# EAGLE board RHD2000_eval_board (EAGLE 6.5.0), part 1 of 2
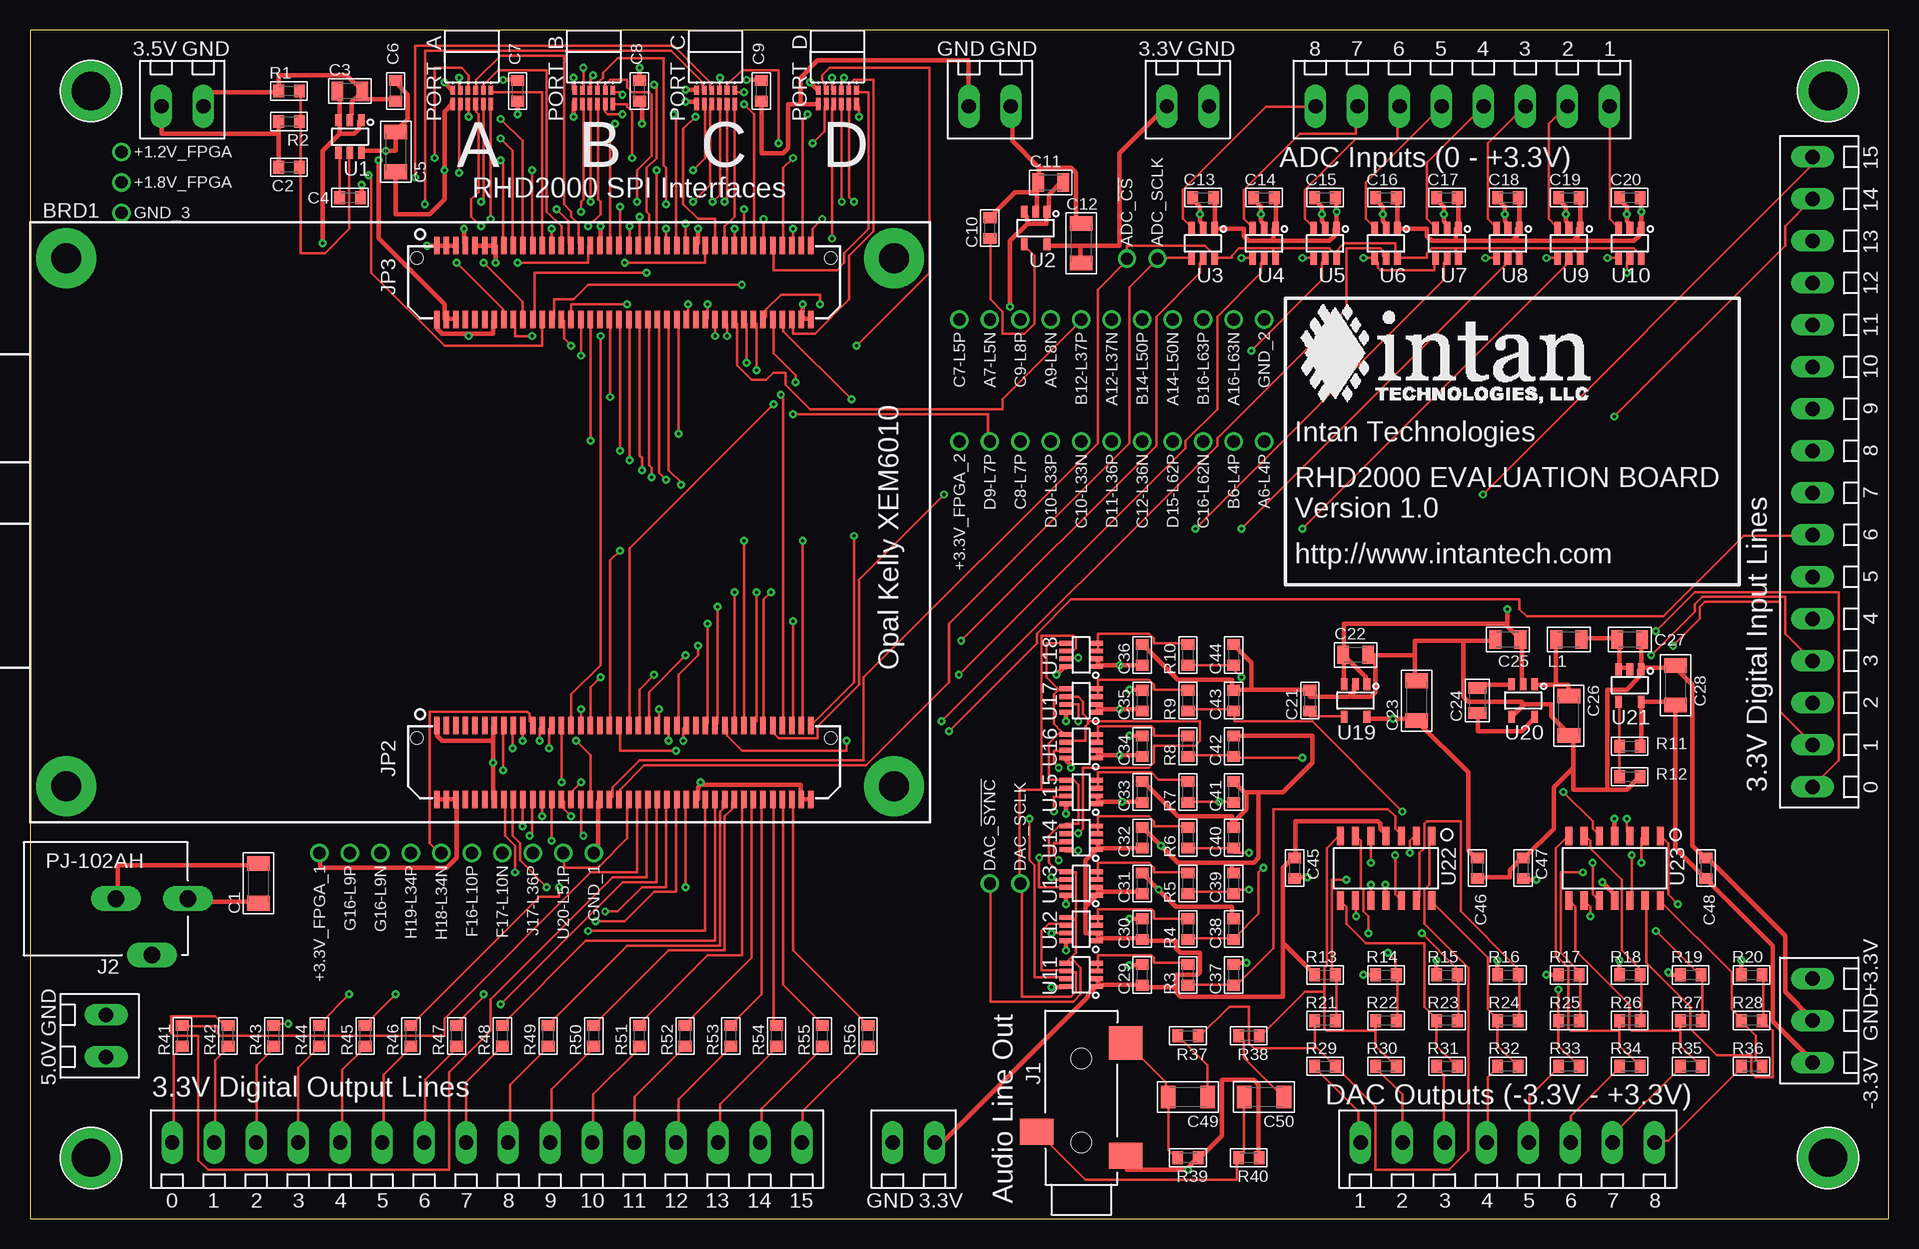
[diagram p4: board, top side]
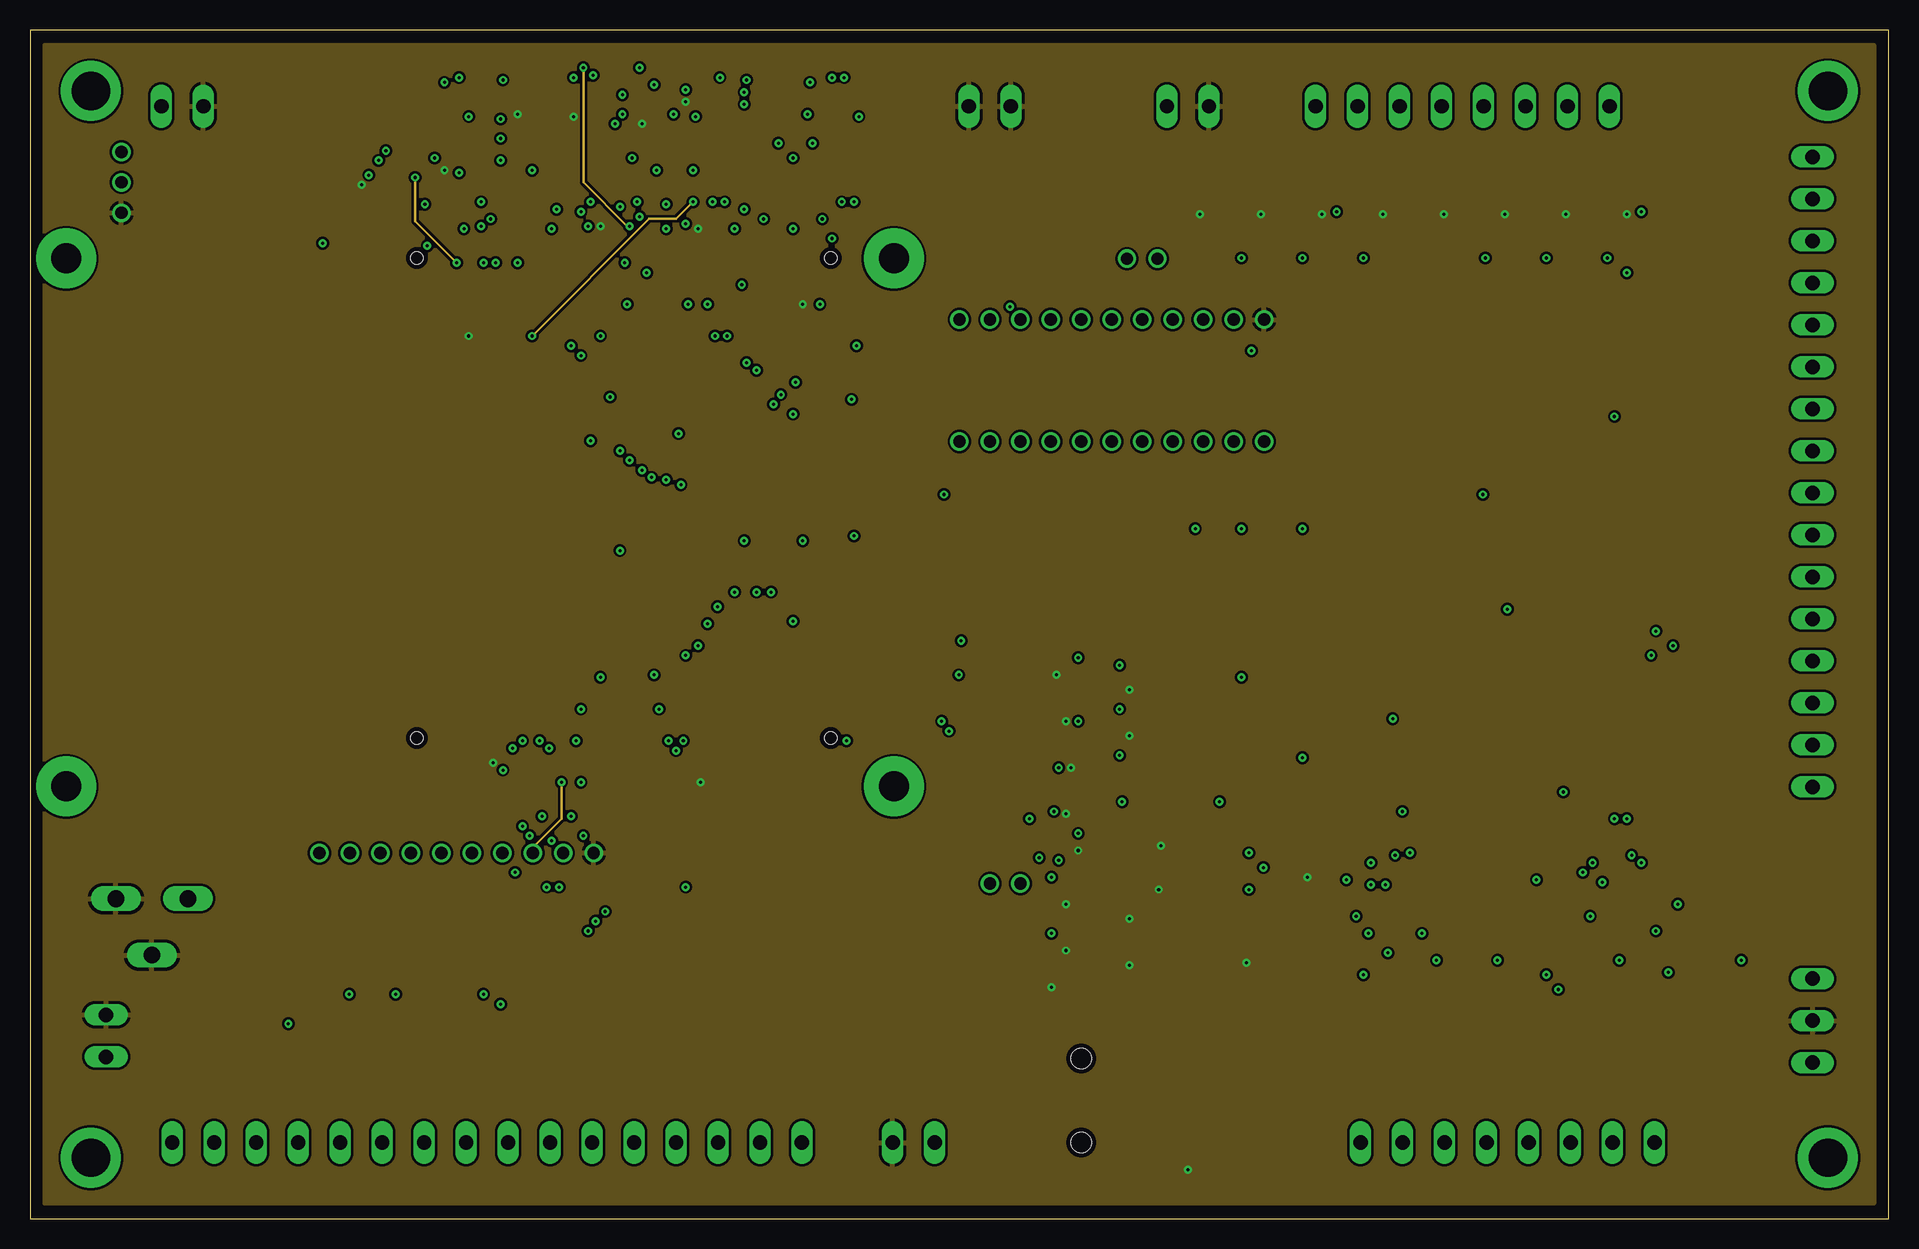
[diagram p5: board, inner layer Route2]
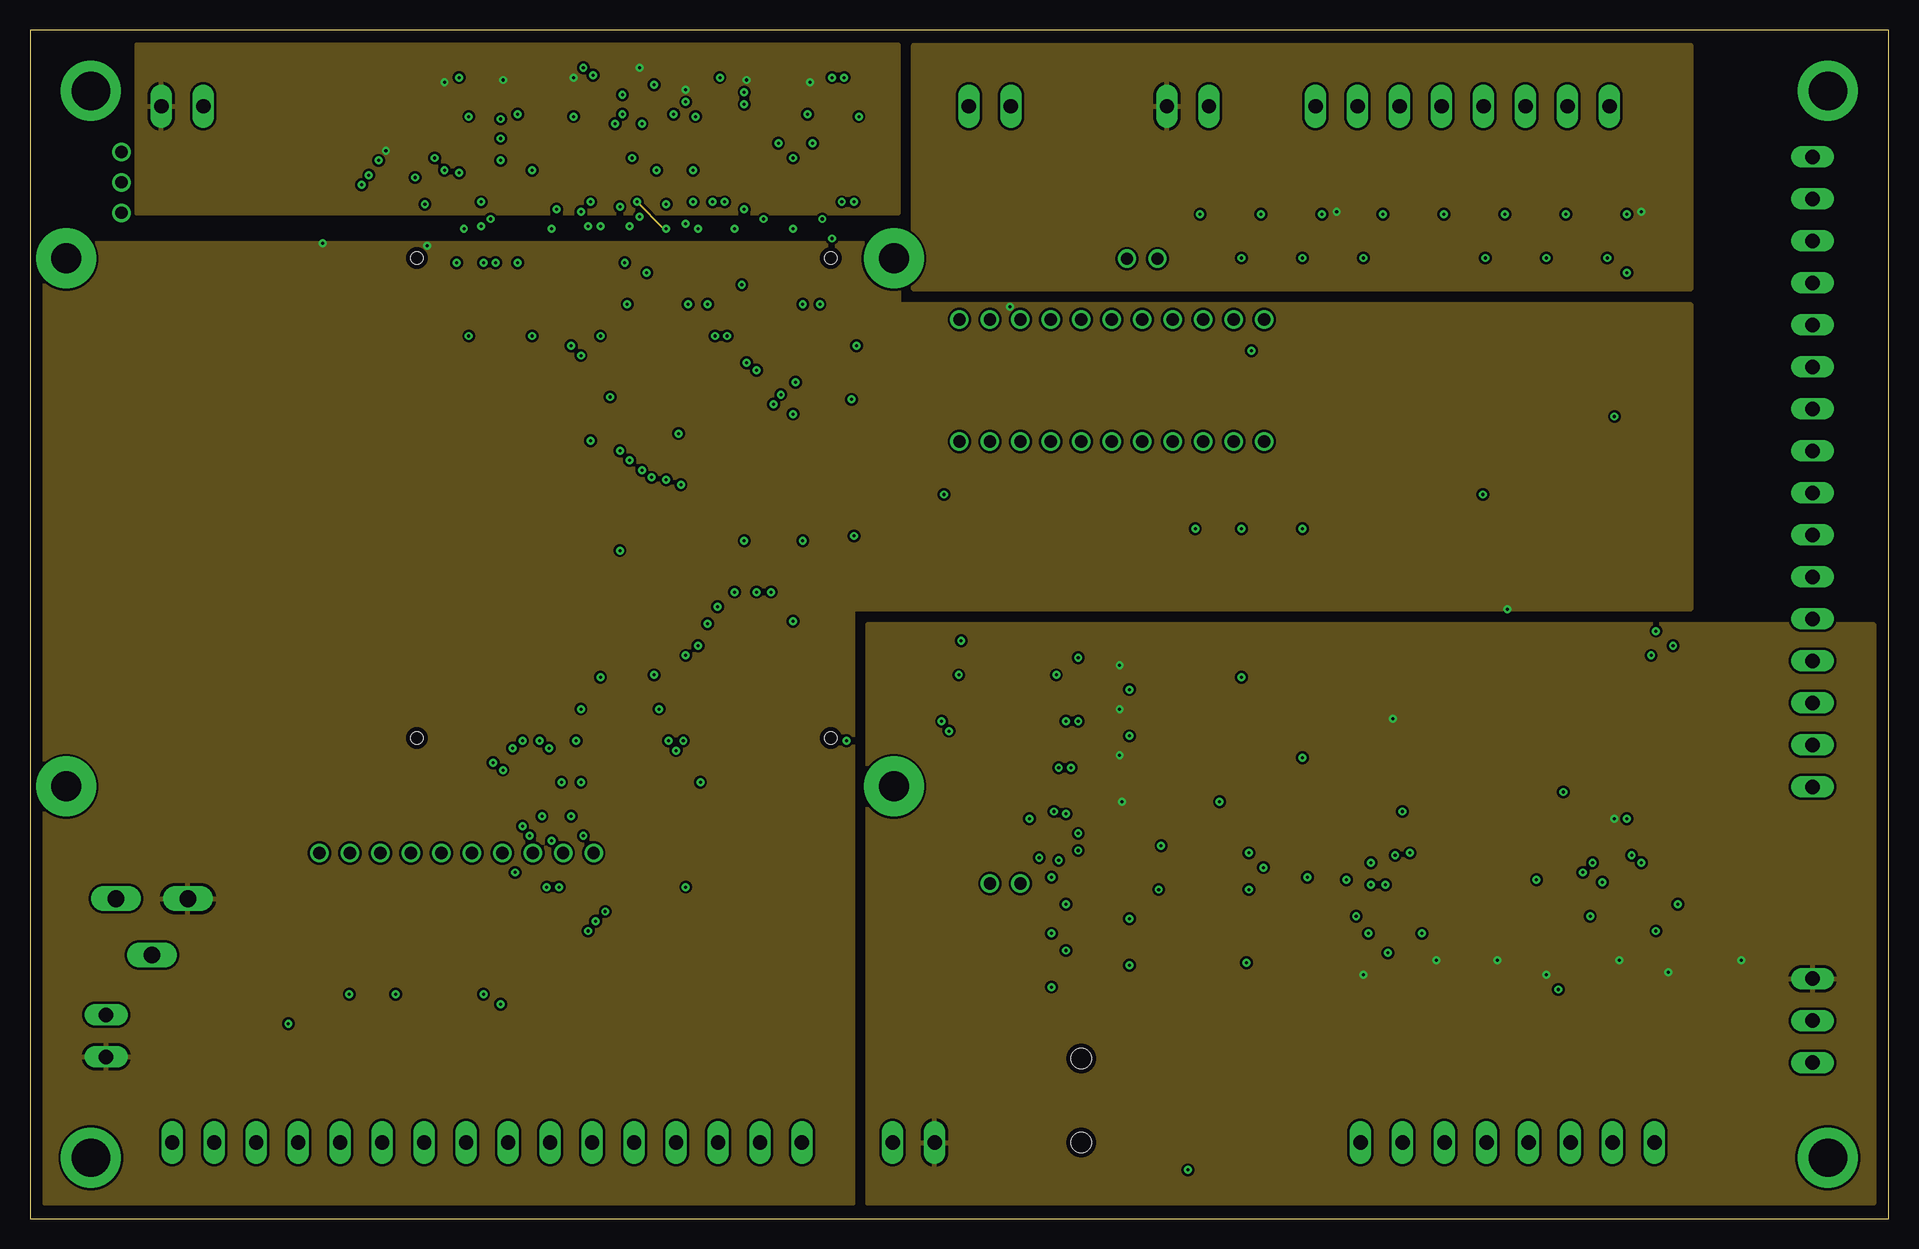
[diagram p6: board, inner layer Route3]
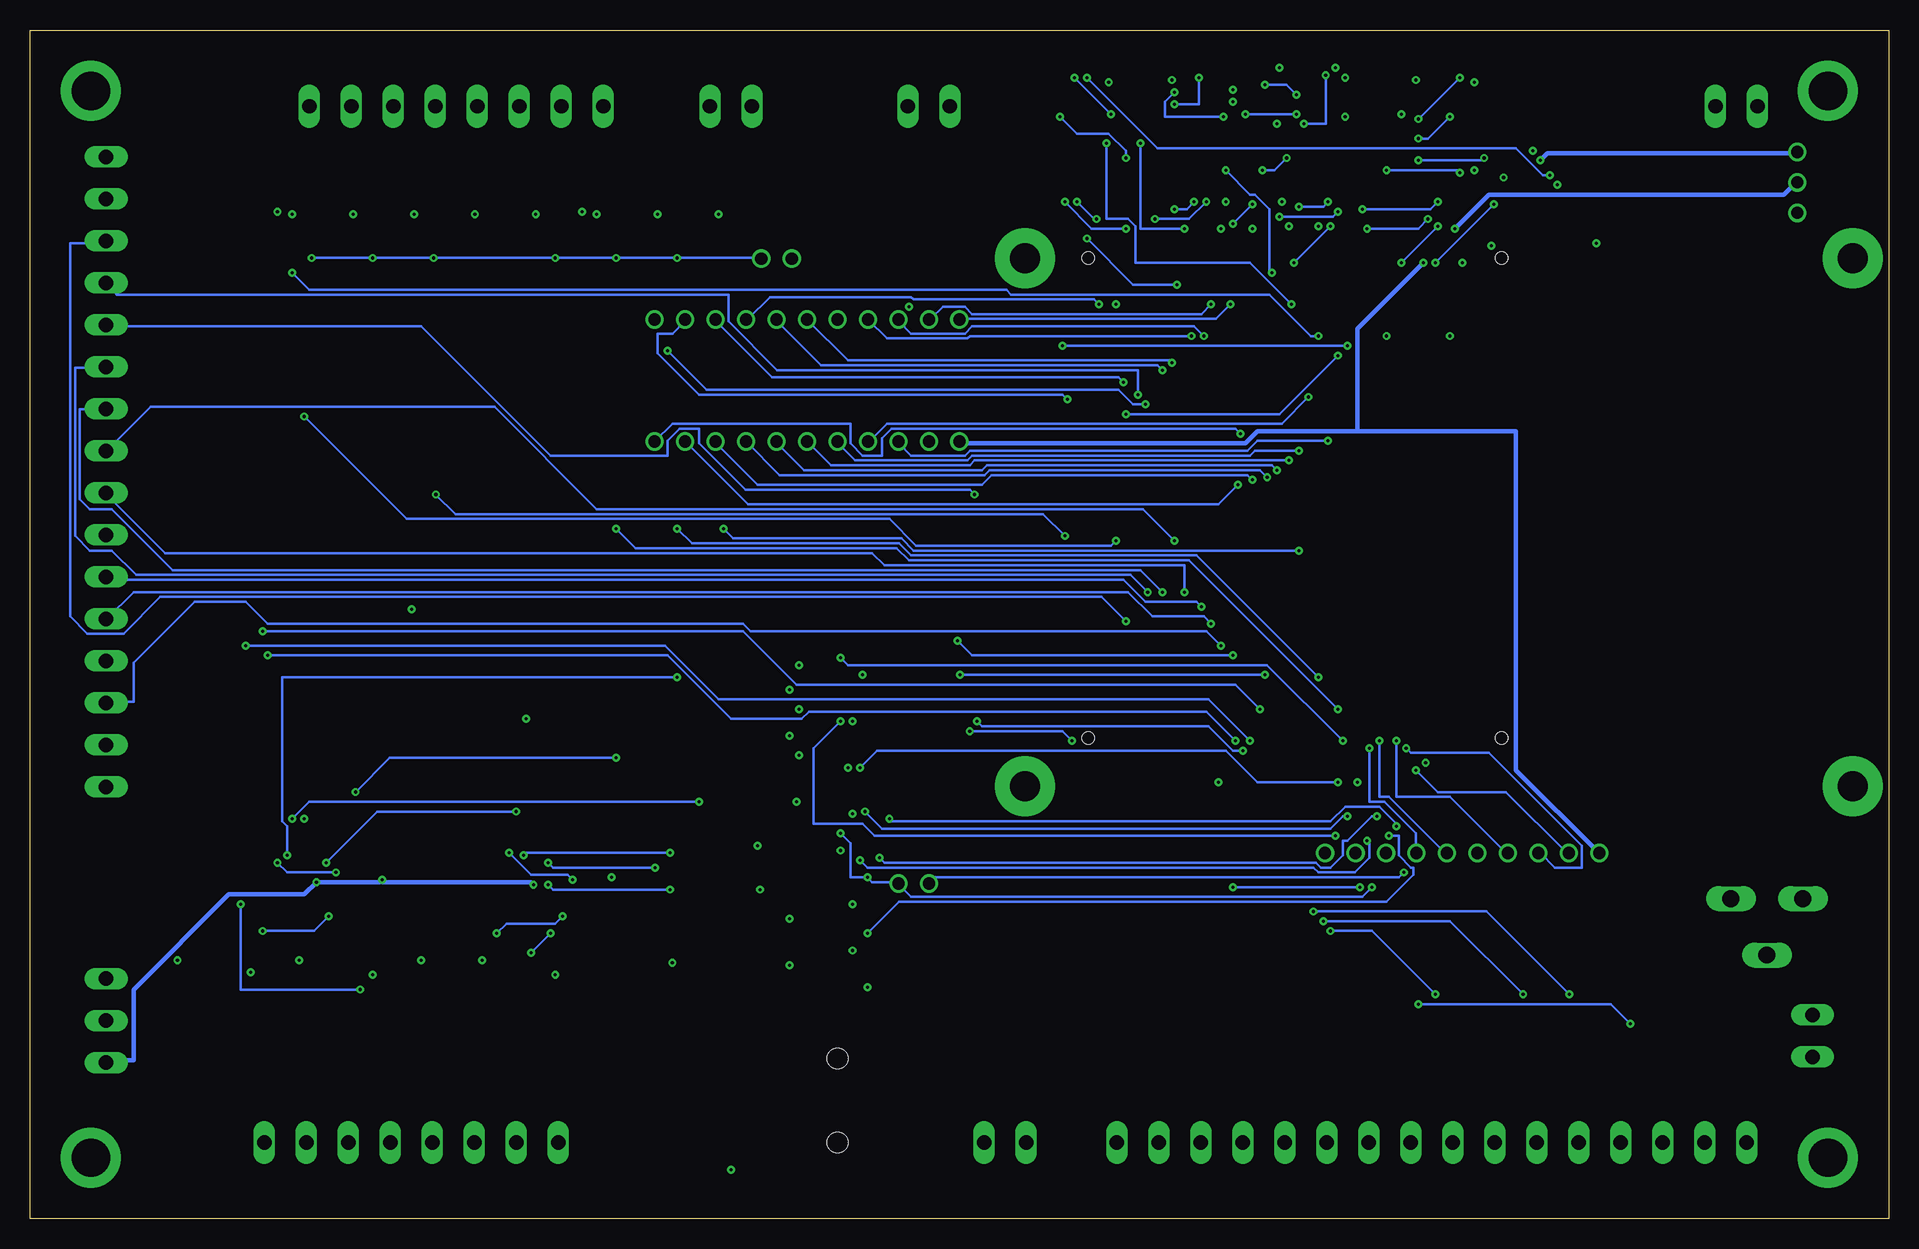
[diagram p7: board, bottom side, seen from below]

Size 154.94 x 99.06 mm. Coordinates in mm from the lower left corner, seen from the top.
Outline: 0,0 154.94,0 154.94,99.06 0,99.06 0,0
Copper layers (1*2+3*16): Top 0.035mm / dielectric 1.5mm / Route2 0.035mm / dielectric 0.15mm / Route3 0.035mm / dielectric 0.2mm / Bottom 0.035mm
Design rules "default": minimum track width 8mil, minimum drill 10mil, track to track 8mil, track to pad 8mil, pad to pad 8mil, via to via 8mil, smd to smd 8mil, copper to edge 15mil, drill to drill 8mil, minimum pad ring 10mil, minimum via ring 8mil, stop-mask expansion 4mil, vias tented up to drill 0mil, thermal gap 10mil
Net classes: 1 power: width 0.381 mm
tRestrict: area 141,33 to 154.9,34.3; area 139.7,33 to 141,50.8; area 137.2,78.7 to 138.4,99.1
vRestrict: area 36.8,85.1 to 68.6,86.9; area 105.4,54.6 to 137.2,56.4; area 105.4,64.8 to 130.8,66.5; area 105.4,61 to 142.2,62.7; area 35.6,87.6 to 38.1,91.4; area 45.7,87.6 to 48.3,91.4; area 55.9,87.6 to 58.4,91.4; area 66,87.6 to 68.6,91.4; area 105.4,58.4 to 120.7,60.2; area 105.7,67.8 to 130.3,76.2

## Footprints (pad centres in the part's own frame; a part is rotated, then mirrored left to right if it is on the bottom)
TERMINAL_BLOCK_3.5MM_16 = drill 1.2 long: 1 -26.25,0; 2 -22.75,0; 3 -19.25,0; 4 -15.75,0; 5 -12.25,0; 6 -8.75,0; 7 -5.25,0; 8 -1.75,0; 9 1.75,0; 10 5.25,0; 11 8.75,0; 12 12.25,0; 13 15.75,0; 14 19.25,0; 15 22.75,0; 16 26.25,0
TESTPOINT = drill 1.016: 1 0,0
TERMINAL_BLOCK_3.5MM_8 = drill 1.2 long: 1 -12.28,0; 2 -8.78,0; 3 -5.28,0; 4 -1.78,0; 5 1.72,0; 6 5.22,0; 7 8.72,0; 8 12.22,0
OPALKELLY_XEM6010 = drill 2.5 pad 5: HOLE_NC_1 3,3; HOLE_NC_2 3,47; HOLE_NC_3 72,3; HOLE_NC_4 72,47 | smd 0.457 x 1.448: JP2-1 33.9,8.086; JP2-2 33.9,1.914; JP2-3 34.7,8.086; JP2-4 34.7,1.914; JP2-5 35.5,8.086; JP2-6 35.5,1.914; JP2-7 36.3,8.086; JP2-8 36.3,1.914; JP2-9 37.1,8.086; JP2-10 37.1,1.914; JP2-11 37.9,8.086; JP2-12 37.9,1.914; JP2-13 38.7,8.086; JP2-14 38.7,1.914; JP2-15 39.5,8.086; JP2-16 39.5,1.914; JP2-17 40.3,8.086; JP2-18 40.3,1.914; JP2-19 41.1,8.086; JP2-20 41.1,1.914; JP2-21 41.9,8.086; JP2-22 41.9,1.914; JP2-23 42.7,8.086; JP2-24 42.7,1.914; JP2-25 43.5,8.086; JP2-26 43.5,1.914; JP2-27 44.3,8.086; JP2-28 44.3,1.914; JP2-29 45.1,8.086; JP2-30 45.1,1.914; JP2-31 45.9,8.086; JP2-32 45.9,1.914; JP2-33 46.7,8.086; JP2-34 46.7,1.914; JP2-35 47.5,8.086; JP2-36 47.5,1.914; JP2-37 48.3,8.086; JP2-38 48.3,1.914; JP2-39 49.1,8.086; JP2-40 49.1,1.914; JP2-41 49.9,8.086; JP2-42 49.9,1.914; JP2-43 50.7,8.086; JP2-44 50.7,1.914; JP2-45 51.5,8.086; JP2-46 51.5,1.914; JP2-47 52.3,8.086; JP2-48 52.3,1.914; JP2-49 53.1,8.086; JP2-50 53.1,1.914; JP2-51 53.9,8.086; JP2-52 53.9,1.914; JP2-53 54.7,8.086; JP2-54 54.7,1.914; JP2-55 55.5,8.086; JP2-56 55.5,1.914; JP2-57 56.3,8.086; JP2-58 56.3,1.914; JP2-59 57.1,8.086; JP2-60 57.1,1.914; JP2-61 57.9,8.086; JP2-62 57.9,1.914; JP2-63 58.7,8.086; JP2-64 58.7,1.914; JP2-65 59.5,8.086; JP2-66 59.5,1.914; JP2-67 60.3,8.086; JP2-68 60.3,1.914; JP2-69 61.1,8.086; JP2-70 61.1,1.914; JP2-71 61.9,8.086; JP2-72 61.9,1.914; JP2-73 62.7,8.086; JP2-74 62.7,1.914; JP2-75 63.5,8.086; JP2-76 63.5,1.914; JP2-77 64.3,8.086; JP2-78 64.3,1.914; JP2-79 65.1,8.086; JP2-80 65.1,1.914; JP3-1 33.9,48.086; JP3-2 33.9,41.914; JP3-3 34.7,48.086; JP3-4 34.7,41.914; JP3-5 35.5,48.086; JP3-6 35.5,41.914; JP3-7 36.3,48.086; JP3-8 36.3,41.914; JP3-9 37.1,48.086; JP3-10 37.1,41.914; JP3-11 37.9,48.086; JP3-12 37.9,41.914; JP3-13 38.7,48.086; JP3-14 38.7,41.914; JP3-15 39.5,48.086; JP3-16 39.5,41.914; JP3-17 40.3,48.086; JP3-18 40.3,41.914; JP3-19 41.1,48.086; JP3-20 41.1,41.914; JP3-21 41.9,48.086; JP3-22 41.9,41.914; JP3-23 42.7,48.086; JP3-24 42.7,41.914; JP3-25 43.5,48.086; JP3-26 43.5,41.914; JP3-27 44.3,48.086; JP3-28 44.3,41.914; JP3-29 45.1,48.086; JP3-30 45.1,41.914; JP3-31 45.9,48.086; JP3-32 45.9,41.914; JP3-33 46.7,48.086; JP3-34 46.7,41.914; JP3-35 47.5,48.086; JP3-36 47.5,41.914; JP3-37 48.3,48.086; JP3-38 48.3,41.914; JP3-39 49.1,48.086; JP3-40 49.1,41.914; JP3-41 49.9,48.086; JP3-42 49.9,41.914; JP3-43 50.7,48.086; JP3-44 50.7,41.914; JP3-45 51.5,48.086; JP3-46 51.5,41.914; JP3-47 52.3,48.086; JP3-48 52.3,41.914; JP3-49 53.1,48.086; JP3-50 53.1,41.914; JP3-51 53.9,48.086; JP3-52 53.9,41.914; JP3-53 54.7,48.086; JP3-54 54.7,41.914; JP3-55 55.5,48.086; JP3-56 55.5,41.914; JP3-57 56.3,48.086; JP3-58 56.3,41.914; JP3-59 57.1,48.086; JP3-60 57.1,41.914; JP3-61 57.9,48.086; JP3-62 57.9,41.914; JP3-63 58.7,48.086; JP3-64 58.7,41.914; JP3-65 59.5,48.086; JP3-66 59.5,41.914; JP3-67 60.3,48.086; JP3-68 60.3,41.914; JP3-69 61.1,48.086; JP3-70 61.1,41.914; JP3-71 61.9,48.086; JP3-72 61.9,41.914; JP3-73 62.7,48.086; JP3-74 62.7,41.914; JP3-75 63.5,48.086; JP3-76 63.5,41.914; JP3-77 64.3,48.086; JP3-78 64.3,41.914; JP3-79 65.1,48.086; JP3-80 65.1,41.914 | hole 1.016: 32.261,47.032; 66.739,47.032; 32.261,7.032; 66.739,7.032
1206 = smd 1.219 x 1.88: 1 -1.651,0; 2 1.651,0
0603 = smd 0.889 x 1.067: 1 -0.864,0; 2 0.864,0
0805 = smd 0.965 x 1.524: 1 -1.041,0; 2 1.041,0
SCREW_HOLE_4-40 = drill 3.2 pad 5: 1 0,0
SJ-3523 = smd 2.2 x 2.8: 1 -1.1,-3.7; 3 0.9,3.7 | smd 2.8 x 2.8: 2 8.3,-3.7 | hole 1.7: 7,0; 0,0
PJ-102AH = drill 1.4 long: 1 0,-3; 2 0,3; 3 -4.7,0
OMNETICS_PZN-12-AA = smd 0.381 x 0.762: B1 1.587,-1.016; B2 0.953,-1.016; B3 0.318,-1.016; B4 -0.318,-1.016; B5 -0.953,-1.016; B6 -1.587,-1.016 | smd 0.381 x 1.016: T1 1.587,-2.159; T2 0.953,-2.159; T3 0.318,-2.159; T4 -0.318,-2.159; T5 -0.953,-2.159; T6 -1.587,-2.159
TERMINAL_BLOCK_3.5MM_3 = drill 1.2 long: + 3.5,0; - -3.5,0; GND 0,0
TERMINAL_BLOCK_3.5MM_2_3.3V = drill 1.2 long: 1 -1.75,0; 2 1.75,0
TERMINAL_BLOCK_3.5MM_2_GND = drill 1.2 long: 1 -1.75,0; 2 1.75,0
TERMINAL_BLOCK_3.5MM_2_5V = drill 1.2 long: 1 -1.75,0; 2 1.75,0
TERMINAL_BLOCK_3.5MM_2_3.5V = drill 1.2 long: 1 -1.75,0; 2 1.75,0
SOT-23-6 = smd 0.55 x 1: 1 -0.95,-1.35; 2 0,-1.35; 3 0.95,-1.35; 4 0.95,1.35; 5 0,1.35; 6 -0.95,1.35
SOT-23-5 = smd 0.55 x 1: 1 -0.95,-1.35; 2 0,-1.35; 3 0.95,-1.35; 4 0.95,1.35; 5 -0.95,1.35
SOT-23-RJ-6 = smd 0.55 x 1: 1 -0.95,-1.3; 2 0,-1.3; 3 0.95,-1.3; 4 0.95,1.3; 5 0,1.3; 6 -0.95,1.3
SOT-23-RJ-8 = smd 0.4 x 1: 1 -0.975,-1.3; 2 -0.325,-1.3; 3 0.325,-1.3; 4 0.975,-1.3; 5 0.975,1.3; 6 0.325,1.3; 7 -0.325,1.3; 8 -0.975,1.3
SOIC-14 = smd 0.6 x 1.55: 1 -3.81,-2.7; 2 -2.54,-2.7; 3 -1.27,-2.7; 4 0,-2.7; 5 1.27,-2.7; 6 2.54,-2.7; 7 3.81,-2.7; 8 3.81,2.7; 9 2.54,2.7; 10 1.27,2.7; 11 0,2.7; 12 -1.27,2.7; 13 -2.54,2.7; 14 -3.81,2.7

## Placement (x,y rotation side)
3.3V_DIGITAL_IN  TERMINAL_BLOCK_16-3.5MM  [TERMINAL_BLOCK_3.5MM_16]  148.59,62.23 90 top
3.3V_DIGITAL_OUT  TERMINAL_BLOCK_16-3.5MM  [TERMINAL_BLOCK_3.5MM_16]  38.1,6.35 0 top
+1.2V_FPGA  TESTPOINT  [TESTPOINT]  7.62,88.9 0 top
+1.8V_FPGA  TESTPOINT  [TESTPOINT]  7.62,86.36 0 top
+3.3V_FPGA_1  TESTPOINT  [TESTPOINT]  24.13,30.48 270 top
+3.3V_FPGA_2  TESTPOINT  [TESTPOINT]  77.47,64.77 270 top
A6-L4P  TESTPOINT  [TESTPOINT]  102.87,64.77 270 top
A7-L5N  TESTPOINT  [TESTPOINT]  80.01,74.93 270 top
A9-L8N  TESTPOINT  [TESTPOINT]  85.09,74.93 270 top
A12-L37N  TESTPOINT  [TESTPOINT]  90.17,74.93 270 top
A14-L50N  TESTPOINT  [TESTPOINT]  95.25,74.93 270 top
A16-L63N  TESTPOINT  [TESTPOINT]  100.33,74.93 270 top
ADC_!CS!  TESTPOINT  [TESTPOINT]  91.44,80.01 90 top
ADC_IN  TERMINAL_BLOCK_8-3.5MM  [TERMINAL_BLOCK_3.5MM_8]  119.38,92.71 180 top
ADC_SCLK  TESTPOINT  [TESTPOINT]  93.98,80.01 90 top
B6-L4P  TESTPOINT  [TESTPOINT]  100.33,64.77 270 top
B12-L37P  TESTPOINT  [TESTPOINT]  87.63,74.93 270 top
B14-L50P  TESTPOINT  [TESTPOINT]  92.71,74.93 270 top
B16-L63P  TESTPOINT  [TESTPOINT]  97.79,74.93 270 top
BRD1  OPALKELLY_XEM6010  [OPALKELLY_XEM6010]  0,33.02 0 top
C1  22u  [1206]  19.05,27.94 90 top
C2  15p  [0603]  21.59,87.63 0 top
C3  1.0u  [0805]  26.67,93.98 0 top
C4  10n  [0603]  26.67,85.09 0 top
C5  22u  [1206]  30.48,88.9 270 top
C6  100n  [0603]  30.48,93.98 270 top
C7  100n  [0603]  40.64,93.98 270 top
C7-L5P  TESTPOINT  [TESTPOINT]  77.47,74.93 270 top
C8  100n  [0603]  50.8,93.98 270 top
C8-L7P  TESTPOINT  [TESTPOINT]  82.55,64.77 270 top
C9  100n  [0603]  60.96,93.98 270 top
C9-L8P  TESTPOINT  [TESTPOINT]  82.55,74.93 270 top
C10  10n  [0603]  80.01,82.55 90 top
C10-L33N  TESTPOINT  [TESTPOINT]  87.63,64.77 270 top
C11  1.0u  [0805]  85.09,86.36 180 top
C12  22u  [1206]  87.63,81.28 90 top
C12-L36N  TESTPOINT  [TESTPOINT]  92.71,64.77 270 top
C13  100n  [0603]  97.79,85.09 180 top
C14  100n  [0603]  102.87,85.09 180 top
C15  100n  [0603]  107.95,85.09 180 top
C16  100n  [0603]  113.03,85.09 180 top
C16-L62N  TESTPOINT  [TESTPOINT]  97.79,64.77 270 top
C17  100n  [0603]  118.11,85.09 180 top
C18  100n  [0603]  123.19,85.09 180 top
C19  100n  [0603]  128.27,85.09 180 top
C20  100n  [0603]  133.35,85.09 180 top
C21  10n  [0603]  106.68,43.18 90 top
C22  1.0u  [0805]  110.49,46.99 0 top
C23  22u  [1206]  115.57,43.18 90 top
C24  1.0u  [0805]  120.65,43.18 90 top
C25  1.0u  [0805]  123.19,48.26 180 top
C26  10u  [1206]  128.27,41.91 270 top
C27  1.0u  [0805]  133.35,48.26 0 top
C28  22u  [1206]  137.16,44.45 90 top
C29  100n  [0603]  92.71,20.32 90 top
C30  100n  [0603]  92.71,24.13 90 top
C31  100n  [0603]  92.71,27.94 90 top
C32  100n  [0603]  92.71,31.75 90 top
C33  100n  [0603]  92.71,35.56 90 top
C34  100n  [0603]  92.71,39.37 90 top
C35  100n  [0603]  92.71,43.18 90 top
C36  100n  [0603]  92.71,46.99 90 top
C37  1n  [0603]  100.33,20.32 90 top
C38  1n  [0603]  100.33,24.13 90 top
C39  1n  [0603]  100.33,27.94 90 top
C40  1n  [0603]  100.33,31.75 90 top
C41  1n  [0603]  100.33,35.56 90 top
C42  1n  [0603]  100.33,39.37 90 top
C43  1n  [0603]  100.33,43.18 90 top
C44  1n  [0603]  100.33,46.99 90 top
C45  100n  [0603]  105.41,29.21 270 top
C46  100n  [0603]  120.65,29.21 270 top
C47  100n  [0603]  124.46,29.21 270 top
C48  100n  [0603]  139.7,29.21 270 top
C49  22u  [1206]  96.52,10.16 180 top
C50  22u  [1206]  102.87,10.16 180 top
D9-L7P  TESTPOINT  [TESTPOINT]  80.01,64.77 270 top
D10-L33P  TESTPOINT  [TESTPOINT]  85.09,64.77 270 top
D11-L36P  TESTPOINT  [TESTPOINT]  90.17,64.77 270 top
D15-L62P  TESTPOINT  [TESTPOINT]  95.25,64.77 270 top
DAC_!SYNC!  TESTPOINT  [TESTPOINT]  80.01,27.94 90 top
DAC_OUT  TERMINAL_BLOCK_8-3.5MM  [TERMINAL_BLOCK_3.5MM_8]  123.19,6.35 0 top
DAC_SCLK  TESTPOINT  [TESTPOINT]  82.55,27.94 90 top
F16-L10P  TESTPOINT  [TESTPOINT]  36.83,30.48 270 top
F17-L10N  TESTPOINT  [TESTPOINT]  39.37,30.48 270 top
G16-L9N  TESTPOINT  [TESTPOINT]  29.21,30.48 270 top
G16-L9P  TESTPOINT  [TESTPOINT]  26.67,30.48 270 top
GND_1  TESTPOINT  [TESTPOINT]  46.99,30.48 270 top
GND_2  TESTPOINT  [TESTPOINT]  102.87,74.93 270 top
GND_3  TESTPOINT  [TESTPOINT]  7.62,83.82 0 top
H1  SCREW_HOLE_4-40  [SCREW_HOLE_4-40]  5.08,93.98 0 top
H2  SCREW_HOLE_4-40  [SCREW_HOLE_4-40]  149.86,93.98 0 top
H3  SCREW_HOLE_4-40  [SCREW_HOLE_4-40]  149.86,5.08 0 top
H4  SCREW_HOLE_4-40  [SCREW_HOLE_4-40]  5.08,5.08 0 top
H18-L34N  TESTPOINT  [TESTPOINT]  34.29,30.48 270 top
H19-L34P  TESTPOINT  [TESTPOINT]  31.75,30.48 270 top
J1  STEREO_JACK_SJ-3523  [SJ-3523]  87.63,6.35 90 top
J2  DC_POWER_JACK-PJ-102AH  [PJ-102AH]  10.16,26.67 90 top
J17-L36P  TESTPOINT  [TESTPOINT]  41.91,30.48 270 top
L1  100n  [0805]  128.27,48.26 0 top
LOGO1  INTAN_LOGO  [INTAN_LOGO]  105.41,67.31 0 top
PORT_A  RHD2000-CABLE-DAQ-SIDE  [OMNETICS_PZN-12-AA]  36.83,95.05 0 top
PORT_B  RHD2000-CABLE-DAQ-SIDE  [OMNETICS_PZN-12-AA]  46.99,95.05 0 top
PORT_C  RHD2000-CABLE-DAQ-SIDE  [OMNETICS_PZN-12-AA]  57.15,95.05 0 top
PORT_D  RHD2000-CABLE-DAQ-SIDE  [OMNETICS_PZN-12-AA]  67.31,95.05 0 top
R1  30.1K  [0603]  21.59,93.98 0 top
R2  56.0K  [0603]  21.59,91.44 180 top
R3  5.6K  [0603]  96.52,20.32 90 top
R4  5.6K  [0603]  96.52,24.13 90 top
R5  5.6K  [0603]  96.52,27.94 90 top
R6  5.6K  [0603]  96.52,31.75 90 top
R7  5.6K  [0603]  96.52,35.56 90 top
R8  5.6K  [0603]  96.52,39.37 90 top
R9  5.6K  [0603]  96.52,43.18 90 top
R10  5.6K  [0603]  96.52,46.99 90 top
R11  64.9K  [0603]  133.35,39.37 0 top
R12  36.0K  [0603]  133.35,36.83 180 top
R13  10k  [0603]  107.95,20.32 0 top
R14  10k  [0603]  113.03,20.32 0 top
R15  10k  [0603]  118.11,20.32 0 top
R16  10k  [0603]  123.19,20.32 0 top
R17  10k  [0603]  128.27,20.32 0 top
R18  10k  [0603]  133.35,20.32 0 top
R19  10k  [0603]  138.43,20.32 0 top
R20  10k  [0603]  143.51,20.32 0 top
R21  10k  [0603]  107.95,16.51 0 top
R22  10k  [0603]  113.03,16.51 0 top
R23  10k  [0603]  118.11,16.51 0 top
R24  10k  [0603]  123.19,16.51 0 top
R25  10k  [0603]  128.27,16.51 0 top
R26  10k  [0603]  133.35,16.51 0 top
R27  10k  [0603]  138.43,16.51 0 top
R28  10k  [0603]  143.51,16.51 0 top
R29  51  [0603]  107.95,12.7 0 top
R30  51  [0603]  113.03,12.7 0 top
R31  51  [0603]  118.11,12.7 0 top
R32  51  [0603]  123.19,12.7 0 top
R33  51  [0603]  128.27,12.7 0 top
R34  51  [0603]  133.35,12.7 0 top
R35  51  [0603]  138.43,12.7 0 top
R36  51  [0603]  143.51,12.7 0 top
R37  100  [0603]  96.52,15.24 180 top
R38  100  [0603]  101.6,15.24 180 top
R39  1.0M  [0603]  96.52,5.08 180 top
R40  1.0M  [0603]  101.6,5.08 180 top
R41  51  [0603]  12.7,15.24 90 top
R42  51  [0603]  16.51,15.24 90 top
R43  51  [0603]  20.32,15.24 90 top
R44  51  [0603]  24.13,15.24 90 top
R45  51  [0603]  27.94,15.24 90 top
R46  51  [0603]  31.75,15.24 90 top
R47  51  [0603]  35.56,15.24 90 top
R48  51  [0603]  39.37,15.24 90 top
R49  51  [0603]  43.18,15.24 90 top
R50  51  [0603]  46.99,15.24 90 top
R51  51  [0603]  50.8,15.24 90 top
R52  51  [0603]  54.61,15.24 90 top
R53  51  [0603]  58.42,15.24 90 top
R54  51  [0603]  62.23,15.24 90 top
R55  51  [0603]  66.04,15.24 90 top
R56  51  [0603]  69.85,15.24 90 top
S1  TERMINAL_BLOCK_3_+/-3.3V  [TERMINAL_BLOCK_3.5MM_3]  148.59,16.51 90 top
S2  TERMINAL_BLOCK_2-3.5MM-3.3V  [TERMINAL_BLOCK_3.5MM_2_3.3V]  96.52,92.71 180 top
S6  TERMINAL_BLOCK_2-3.5MM-3.3V  [TERMINAL_BLOCK_3.5MM_2_3.3V]  73.66,6.35 0 top
S8  TERMINAL_BLOCK_2-3.5MM-GND  [TERMINAL_BLOCK_3.5MM_2_GND]  80.01,92.71 180 top
S9  TERMINAL_BLOCK_2-3.5MM-5V  [TERMINAL_BLOCK_3.5MM_2_5V]  6.35,15.24 270 top
S10  TERMINAL_BLOCK_2-3.5MM-3.5V  [TERMINAL_BLOCK_3.5MM_2_3.5V]  12.7,92.71 180 top
U1  TPS79301  [SOT-23-6]  26.67,90.17 180 top
U2  TPS79333  [SOT-23-5]  83.82,82.55 180 top
U3  AD7680-SOT-23  [SOT-23-RJ-6]  97.79,81.28 180 top
U4  AD7680-SOT-23  [SOT-23-RJ-6]  102.87,81.28 180 top
U5  AD7680-SOT-23  [SOT-23-RJ-6]  107.95,81.28 180 top
U6  AD7680-SOT-23  [SOT-23-RJ-6]  113.03,81.28 180 top
U7  AD7680-SOT-23  [SOT-23-RJ-6]  118.11,81.28 180 top
U8  AD7680-SOT-23  [SOT-23-RJ-6]  123.19,81.28 180 top
U9  AD7680-SOT-23  [SOT-23-RJ-6]  128.27,81.28 180 top
U10  AD7680-SOT-23  [SOT-23-RJ-6]  133.35,81.28 180 top
U11  AD5662-SOT-23  [SOT-23-RJ-8]  87.63,20.32 90 top
U12  AD5662-SOT-23  [SOT-23-RJ-8]  87.63,24.13 90 top
U13  AD5662-SOT-23  [SOT-23-RJ-8]  87.63,27.94 90 top
U14  AD5662-SOT-23  [SOT-23-RJ-8]  87.63,31.75 90 top
U15  AD5662-SOT-23  [SOT-23-RJ-8]  87.63,35.56 90 top
U16  AD5662-SOT-23  [SOT-23-RJ-8]  87.63,39.37 90 top
U17  AD5662-SOT-23  [SOT-23-RJ-8]  87.63,43.18 90 top
U18  AD5662-SOT-23  [SOT-23-RJ-8]  87.63,46.99 90 top
U19  TPS79333  [SOT-23-5]  110.49,43.18 180 top
U20  TPS60403  [SOT-23-5]  124.46,43.18 180 top
U20-L51P  TESTPOINT  [TESTPOINT]  44.45,30.48 270 top
U21  TPS72301  [SOT-23-5]  133.35,44.45 180 top
U22  OPA4170_SO14  [SOIC-14]  113.03,29.21 180 top
U23  OPA4170_SO14  [SOIC-14]  132.08,29.21 180 top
